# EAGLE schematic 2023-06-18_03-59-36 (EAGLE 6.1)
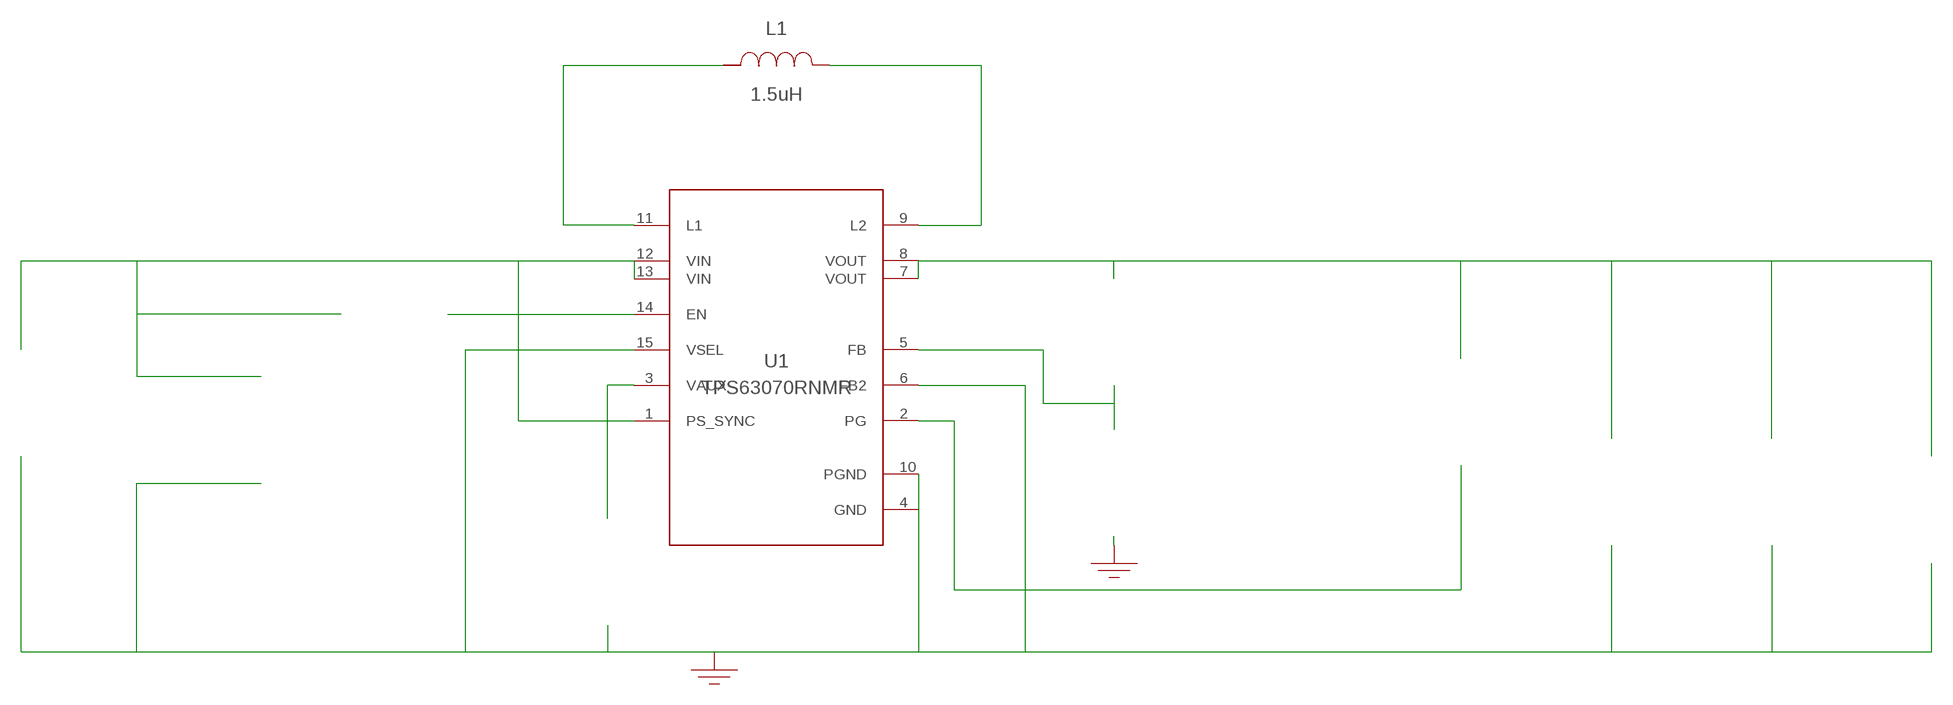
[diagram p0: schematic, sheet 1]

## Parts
CAUX  100nF  GRM155R71C104KA88DGRM155R71C104KA88D  [0402]  (not placed on a sheet)
CIN  22uF  GRM32ER61E226KE15LGRM32ER61E226KE15L  [1210]  (not placed on a sheet)
CIN_2  22uF  GRM32ER61E226KE15LGRM32ER61E226KE15L  [1210]  (not placed on a sheet)
COUT  47uF  GRM31CR60J476KE19LGRM31CR60J476KE19L  [1206_190]  (not placed on a sheet)
COUTX  10uF  GRM188R60J106ME47DGRM188R60J106ME47D  [0603]  (not placed on a sheet)
GND  WB_GND  WB_GNDWB_GND  [WB_GND]
GND2  WB_GND  WB_GNDWB_GND  [WB_GND]
IOUT  WB_CURRENT_LOAD  WB_CURRENT_LOADWB_CURRENT_LOAD  [WB_CURRENT_LOAD]  (not placed on a sheet)
L1  1.5uH  SRN8040-1R5YSRN8040-1R5Y  [SRN8040]
RENABLE  10k  RC0201FR-0710KLRC0201FR-0710KL  [0201]  (not placed on a sheet)
RFBB  100k  RC0603FR-07100KLRC0603FR-07100KL  [0603]  (not placed on a sheet)
RFBT  309k  RC0603FR-07309KLRC0603FR-07309KL  [0603]  (not placed on a sheet)
RPGOOD  100k  CRCW0603100KFKEACRCW0603100KFKEA  [0603]  (not placed on a sheet)
U1  TPS63070RNMR  TPS63070RNMRTPS63070RNMR  [RNM0015A]
VIN  WB_BATTERY  WB_BATTERYWB_BATTERY  [WB_BATTERY]  (not placed on a sheet)
Unconnected: CAUX.1 CAUX.2 CIN.1 CIN.2 CIN_2.1 CIN_2.2 COUT.1 COUT.2 COUTX.1 COUTX.2 GND2.1 GND.1 IOUT.1(+) IOUT.2(-) L1.1 L1.2 RENABLE.1 RENABLE.2 RFBB.1 RFBB.2 RFBT.1 RFBT.2 RPGOOD.1 RPGOOD.2 U1.1(PS_SYNC) U1.2(PG) U1.3(VAUX) U1.5(FB) U1.6(FB2) U1.9(L2) U1.11(L1) U1.14(EN) U1.15(VSEL) VIN.1(+) VIN.2(-)

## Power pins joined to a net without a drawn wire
GND: U1.4(GND)
PGND: U1.10(PGND)
VIN: U1.12(VIN) U1.13(VIN)
VOUT: U1.7(VOUT) U1.8(VOUT)

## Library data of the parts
CAUX = AcceleratedDesigns_Lib:GRM155R71C104KA88D; Manufacturer_Part_Number: GRM155R71C104KA88D; Vendor: MuRata
CIN CIN_2 = AcceleratedDesigns_Lib:GRM32ER61E226KE15L; Manufacturer_Part_Number: GRM32ER61E226KE15L; Vendor: MuRata
COUT = AcceleratedDesigns_Lib:GRM31CR60J476KE19L; Manufacturer_Part_Number: GRM31CR60J476KE19L; Vendor: MuRata
COUTX = AcceleratedDesigns_Lib:GRM188R60J106ME47D; Manufacturer_Part_Number: GRM188R60J106ME47D; Vendor: MuRata
GND GND2 = AcceleratedDesigns_Lib:WB_GND; Manufacturer_Part_Number: WB_GND
IOUT = AcceleratedDesigns_Lib:WB_CURRENT_LOAD; Manufacturer_Part_Number: WB_CURRENT_LOAD
L1 = AcceleratedDesigns_Lib:SRN8040-1R5Y; Manufacturer_Part_Number: SRN8040-1R5Y; Vendor: Bourns
RENABLE = AcceleratedDesigns_Lib:RC0201FR-0710KL; Manufacturer_Part_Number: RC0201FR-0710KL; Vendor: Yageo America
RFBB = AcceleratedDesigns_Lib:RC0603FR-07100KL; Manufacturer_Part_Number: RC0603FR-07100KL; Vendor: Yageo America
RFBT = AcceleratedDesigns_Lib:RC0603FR-07309KL; Manufacturer_Part_Number: RC0603FR-07309KL; Vendor: Yageo America
RPGOOD = AcceleratedDesigns_Lib:CRCW0603100KFKEA; Manufacturer_Part_Number: CRCW0603100KFKEA; Vendor: Vishay-Dale
U1 = AcceleratedDesigns_Lib:TPS63070RNMR; Manufacturer_Part_Number: TPS63070RNMR
VIN = AcceleratedDesigns_Lib:WB_BATTERY; Manufacturer_Part_Number: WB_BATTERY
